(* Logix 5000 AddOnInstructionDefinition export Banner_DFG2_DFG3_Param_v4; software revision 33.00 *)

TYPE Banner_DFG2_DFG3_RD_v4 :   // UDT with all of the Read only parameters for DFG2 or DFG3.
STRUCT
   Master_Cycle_Time : INT;
   Min_Cycle_Time : INT;
   M_Sequence_Capability : INT;
   IO_Link_Version_ID : INT;
   Process_Data_Input_Length : INT;
   Process_Data_Output_Length : INT;
   Combined_Vendor_ID : DINT;   // IO-Link Vendor ID
   Vendor_ID1 : INT;
   Vendor_ID2 : INT;
   Combined_Device_ID : DINT;   // IO-Link Device ID
   Device_ID1 : INT;
   Device_ID2 : INT;
   Device_ID3 : INT;
   Serial_Number : STRING;
   Teach_State : SINT;   // 0 =IDLE, 1 = SP1 Success, 4 = Wait for Command, 5 = Busy, 7 = Error
   SP1_TP1 : SINT;   // 0 = Teach point 1 not taught or not successful, 1 = Teach point 1 was successful
   SP1_TP2 : SINT;   // 0 = Teach point 2 not taught or not successful, 1 = Teach point 2 was successful
   SP2_TP1 : SINT;   // 0 = Teach point 2 not taught or not successful, 1 = Teach point 2 was successful
   SP2_TP2 : SINT;   // 0 = Teach point 2 not taught or not successful, 1 = Teach point 2 was successful
   BDC1_Lower_Hysteresis : DINT;
   BDC1_Lower_Threshold : DINT;
   BDC1_Reference : DINT;
   BDC1_Upper_Threshold : DINT;
   BDC1_Upper_Hysteresis : DINT;
   BDC1_Output_State : SINT;   // 0 = Inactive, 1 = Active.
   BDC1_Alarm_State : SINT;   // 0 = No Alarm, 1 = Threshold Warning, 2 = Threshold Alarm.
   BDC2_Lower_Hysteresis : DINT;
   BDC2_Lower_Threshold : DINT;
   BDC2_Reference : DINT;
   BDC2_Upper_Threshold : DINT;
   BDC2_Upper_Hysteresis : DINT;
   BDC2_Output_State : SINT;   // 0 = Inactive, 1 = Active.
   BDC2_Alarm_State : SINT;   // 0 = No Alarm, 1 = Threshold Warning, 2 = Threshold Alarm.
END_STRUCT
END_TYPE

TYPE Banner_DFG2_DFG3_v4 :   // UDT with all of the parameters needed to work with a Banner DF-G2 or DF-G3 IO-Link Sensor.
STRUCT
   Initial_Global_Read : BOOL;   // Determines if all of the IO-Link data has been read into the PLC yet
   Command : INT;   // Value placed in here will activate a read or write to a specifc IO-Link Index
   DFG_Model : SINT;   // 2 = DF-G2, 3 = DF-G3
   Read_Data : Banner_DFG2_DFG3_RD_v4;
   Write_Data : Banner_DFG2_DFG3_WD_v4;
   Archive_Data : Banner_DFG2_DFG3_WD_v4;
   Reset : BOOL;   // Resets AOI. This will force a complete parameter read of the sensor.
END_STRUCT
END_TYPE

TYPE Banner_DFG2_DFG3_WD_v4 :   // UDT with all of the Write only parameters for DFG2 or DFG3.
STRUCT
   System_Command : INT;   // See IODD file for list of commands that can be activated via the System Command interface
   Parameter_Access_Lock : SINT;   // Write access to all read/write parameters is block when this bit is ON.
   Data_Storage_Lock : SINT;   // Data storage mechanism is inhibited when bit is ON.
   Local_Parameterization_Lock : SINT;   // Parameteriation via local control elementes is inhibited.
   Local_User_Interface_Lock : SINT;   // Operation of the hmi on the device is disabled.
   Teach_Channel : INT;   // 0 = Default, 1 = BDC1, 2 = BDC2
   BDC1_Setpoint_SP1 : DINT;   // Switch point value
   BDC1_Setpoint_SP2 : DINT;   // Unused
   BDC1_Swithpoint_Logic : INT;   // 0 = Light Operate, 1 = Dark Operate
   BDC1_BDC_Mode : INT;   // 1 = Single Point, 128 = Window Set, 129 = Light Set, 130 = Dark Set
   BDC1_Hysteresis : DINT;   // User selectable Hysteresis. 0 = 1.0x, 1 = 1.5x, and 2 = 2.5x.
   BDC2_Setpoint_SP1 : DINT;   // Switch point value
   BDC2_Setpoint_SP2 : DINT;   // Unused
   BDC2_Switchpoint_Logic : INT;   // 0 = Light Operate, 1 = Dark Operate
   BDC2_BDC_Mode : INT;   // 1 = Single Point, 128 = Window Set, 129 = Light Set, 130 = Dark Set
   BDC2_Hysteresis : DINT;   // User selectable Hysteresis. 0 = 1.0x, 1 = 1.5x, and 2 = 2.5x.
   Response_Speed : INT;   // See IODD file for allowable values.
   Gain : INT;   // 0 = Fixed Gain, 1 = Auto Gain
   Gain_Level : INT;   // See IODD file for allowable values.
   AutoThreshold_Response_Time : INT;   // Used in Light, Dark, or Window Set modes only. 12 = 2.5 s, 13 = 5.0 s, 14 = 10 s, and 15 = 20 s.
   Process_Data_Filter_Update_Time : DINT;   // Amount of time to collect averaged sample for process data.
   Signal_Threshold_Readout : INT;   // 0 = Numeric, 1 = Percentage.
   ECO_Mode : INT;   // Dims the display to reduce current consumption. 0 = Disabled, 1 = Enabled.
   Display_Orientation : INT;   // 0 = Normal, 1 = Flipped.
   Secondary_Output_Function : INT;   // 0 = Independent Output, 1 = Complimentary Output, 2 = Health Output, 3 = Remote Set Input, 4 = Master, 5 = Slave, 6 = LED Off, 7 = LED On, 8 = Gate.
   Slave_Numder : INT;   // Total slaves presetn if in master mode. Slave Address if configured as slave. 1 to 6.
   BDC1_Delay_Mode : INT;   // 0 = Disabled, 1 = Off - On Delay, 2 = Off Oneshot, 3 = On Oneshot
   BDC1_Delay_Timer1 : DINT;   // 0 to 9999. Off delay or On/Off Oneshot time. If configured in Oneshot mode, this parameter wil have a minimum value of 1 ms.
   BDC1_Delay_Timer2 : DINT;   // 0 to 9999. On delay time or additional delay time. In off/on delay mode, this parameter will be the on delay.
   BDC1_Teach_Selection : INT;   // 0 = Two-Point Teach, 1 = Dynamic Teach, 2 = Window Teach, 3 = Light Set, 4 = Dark Set, 5 = Cal Set
   BDC1_Offset_Percent : DINT;   // Used during the Window, Light, or Dark Set methods. The threshold(s) are positioned in a programmable % offset from the taught condition.
   BDC1_Auto_Thresholding : INT;   // 0 = Disabled, 1 = Enabled. The auto thresholds algorithm continuously tracks slow changes in the taught condition(s) and optimizes the threshold(s) to provide for reliable sensing.
   BDC2_Delay_Mode : INT;   // 0 = Disabled, 1 = Off - On Delay, 2 = Off Oneshot, 3 = On Oneshot
   BDC2_Delay_Timer1 : DINT;   // 0 to 9999. Off delay or On/Off Oneshot time. If configured in Oneshot mode, this parameter wil have a minimum value of 1 ms.
   BDC2_Delay_Timer2 : DINT;   // 0 to 9999. On delay time or additional delay time. In off/on delay mode, this parameter will be the on delay.
   BDC2_Teach_Selection : INT;   // 0 = Two-Point Teach, 1 = Dynamic Teach, 2 = Window Teach, 3 = Light Set, 4 = Dark Set, 5 = Cal Set
   BDC2_Offset_Percent : DINT;   // Used during the Window, Light, or Dark Set methods. The threshold(s) are positioned in a programmable % offset from the taught condition.
   BDC2_Auto_Thresholding : INT;   // 0 = Disabled, 1 = Enabled. The auto thresholds algorithm continuously tracks slow changes in the taught condition(s) and optimizes the threshold(s) to provide for reliable sensing.
END_STRUCT
END_TYPE

TYPE Banner_IOL_Port_v4 :   // UDT that has all of the data items necessary to communicate with a specific Port on a IO-Link Master
STRUCT
   Port_Controlled : INT;   // Each bit represents a port on an IO-Link Master. Set to 1 to tell AOI to control that port.
   Port_Activate : INT;   // Each bit represents a port on an IO-Link Master. When ON that port will process any commands in queue.
   Port_Read : INT;   // Each bit represents a port on an IO-Link Master. Used to determine when device AOI has requested a Read command.
   Port_Write : INT;   // Each bit represents a port on an IO-Link Master. Used to determine when device AOI has requested a Write command.
   Port_RW_Complete : INT;   // Each bit represents a port on an IO-Link Master. Tells device AOI that Read or Write request has been completed.
   Port_Device_Read : INT;
   Data_Transfer : SINT[190];   // Array to transfer data from IO-Master to device AOIs.
END_STRUCT
END_TYPE

ADD_ON_INSTRUCTION Banner_DFG2_DFG3_Param_v4   (* revision 4.1, vendor Banner Engineering *)
// AOI to read and write parameter data to an IO-Link Df-G2 or DF-G3.
VAR_IN_OUT
   DFG2_DFG3 : Banner_DFG2_DFG3_v4; {required}
   Port_Data : Banner_IOL_Port_v4; {required}
END_VAR
VAR_INPUT
   Port : DINT; {required}
END_VAR
VAR
   Local_Control : DINT; {access None}
   Global_Read_Command_Value : INT; {access None}
   Global_Write_Command_Value : INT; {access None}
   Error_Generated : BOOL; {access None}
   Command_Being_Processed : BOOL; {access None}
   Update_Archive : BOOL; {access None}
   Index_Write_Inprocess : DINT; {access None}
   Index_Write_Control : DINT; {access None}
   Inprocess_Index : DINT; {access None}
END_VAR

ROUTINE Logic   (* ladder *)
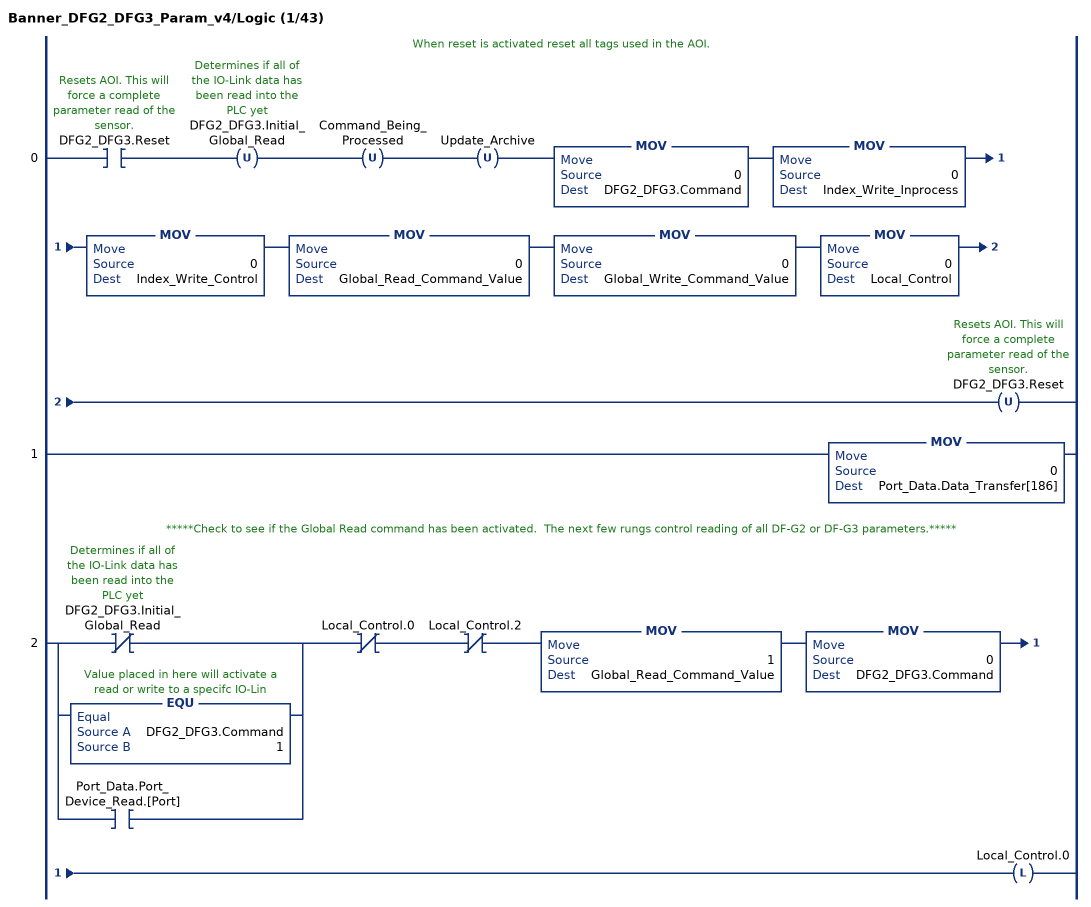
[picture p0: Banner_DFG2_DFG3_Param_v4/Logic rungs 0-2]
   // When reset is activated reset all tags used in the AOI.
   0: XIC(DFG2_DFG3.Reset)OTU(DFG2_DFG3.Initial_Global_Read)OTU(Command_Being_Processed)OTU(Update_Archive)MOV(0,DFG2_DFG3.Command)MOV(0,Index_Write_Inprocess)MOV(0,Index_Write_Control)MOV(0,Global_Read_Command_Value)MOV(0,Global_Write_Command_Value)MOV(0,Local_Control)OTU(DFG2_DFG3.Reset);
   1: MOV(0,Port_Data.Data_Transfer[186]);
   // *****Check to see if the Global Read command has been activated.  The next few rungs control reading of all DF-G2 or DF-G3 parameters.*****
   2: [XIO(DFG2_DFG3.Initial_Global_Read) ,EQU(DFG2_DFG3.Command,1) ,XIC(Port_Data.Port_Device_Read.[Port]) ]XIO(Local_Control.0)XIO(Local_Control.2)MOV(1,Global_Read_Command_Value)MOV(0,DFG2_DFG3.Command)OTL(Local_Control.0);
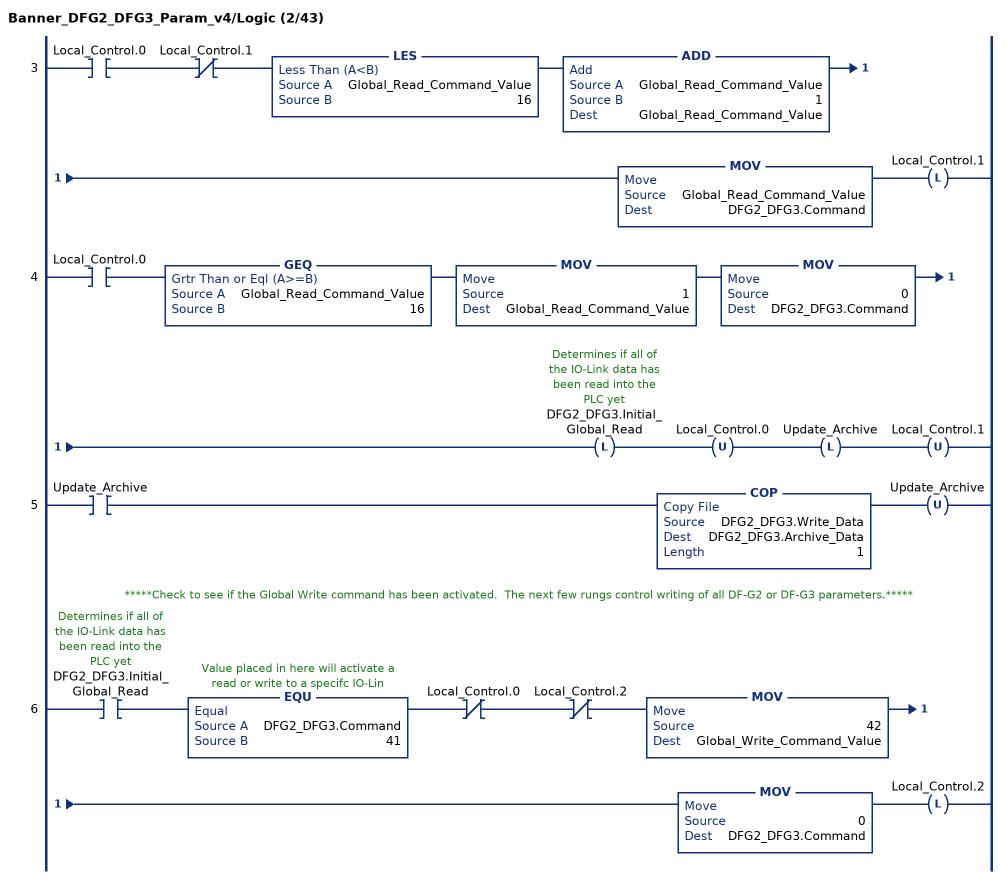
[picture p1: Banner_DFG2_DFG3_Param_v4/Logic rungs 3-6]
   3: XIC(Local_Control.0)XIO(Local_Control.1)LES(Global_Read_Command_Value,16)ADD(Global_Read_Command_Value,1,Global_Read_Command_Value)MOV(Global_Read_Command_Value,DFG2_DFG3.Command)OTL(Local_Control.1);
   4: XIC(Local_Control.0)GEQ(Global_Read_Command_Value,16)MOV(1,Global_Read_Command_Value)MOV(0,DFG2_DFG3.Command)OTL(DFG2_DFG3.Initial_Global_Read)OTU(Local_Control.0)OTL(Update_Archive)OTU(Local_Control.1);
   5: XIC(Update_Archive)COP(DFG2_DFG3.Write_Data,DFG2_DFG3.Archive_Data,1)OTU(Update_Archive);
   // *****Check to see if the Global Write command has been activated.  The next few rungs control writing of all DF-G2 or DF-G3 parameters.*****
   6: XIC(DFG2_DFG3.Initial_Global_Read)EQU(DFG2_DFG3.Command,41)XIO(Local_Control.0)XIO(Local_Control.2)MOV(42,Global_Write_Command_Value)MOV(0,DFG2_DFG3.Command)OTL(Local_Control.2);
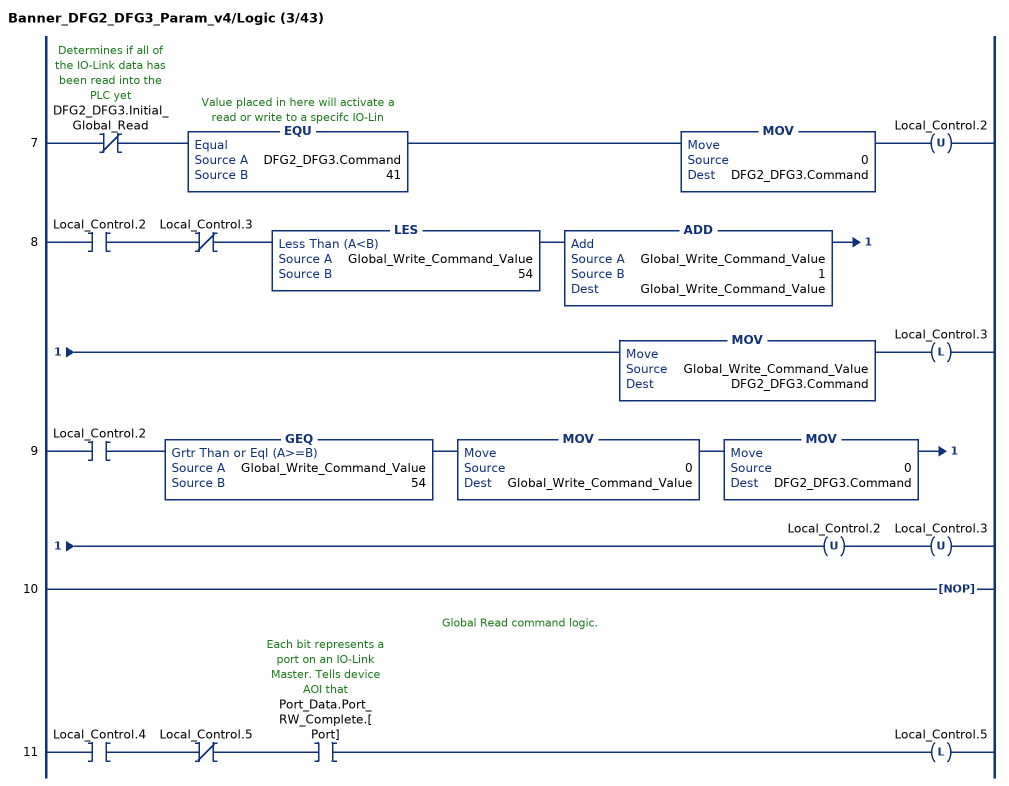
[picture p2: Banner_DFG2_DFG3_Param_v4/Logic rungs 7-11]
   7: XIO(DFG2_DFG3.Initial_Global_Read)EQU(DFG2_DFG3.Command,41)MOV(0,DFG2_DFG3.Command)OTU(Local_Control.2);
   8: XIC(Local_Control.2)XIO(Local_Control.3)LES(Global_Write_Command_Value,54)ADD(Global_Write_Command_Value,1,Global_Write_Command_Value)MOV(Global_Write_Command_Value,DFG2_DFG3.Command)OTL(Local_Control.3);
   9: XIC(Local_Control.2)GEQ(Global_Write_Command_Value,54)MOV(0,Global_Write_Command_Value)MOV(0,DFG2_DFG3.Command)OTU(Local_Control.2)OTU(Local_Control.3);
   10: NOP();
   // Global Read command logic.
   11: XIC(Local_Control.4)XIO(Local_Control.5)XIC(Port_Data.Port_RW_Complete.[Port])OTL(Local_Control.5);
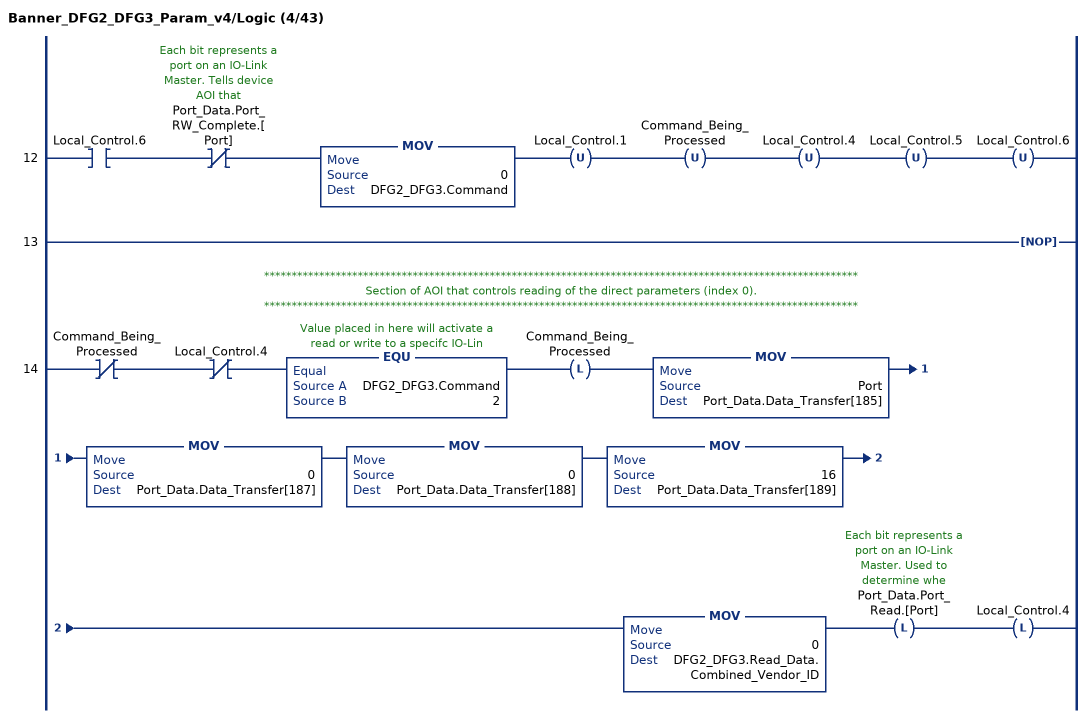
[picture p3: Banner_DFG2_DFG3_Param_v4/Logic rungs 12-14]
   12: XIC(Local_Control.6)XIO(Port_Data.Port_RW_Complete.[Port])MOV(0,DFG2_DFG3.Command)OTU(Local_Control.1)OTU(Command_Being_Processed)OTU(Local_Control.4)OTU(Local_Control.5)OTU(Local_Control.6);
   13: NOP();
   // ************************************************************************************************************
   // Section of AOI that controls reading of the direct parameters (index 0).
   // ************************************************************************************************************
   14: XIO(Command_Being_Processed)XIO(Local_Control.4)EQU(DFG2_DFG3.Command,2)OTL(Command_Being_Processed)MOV(Port,Port_Data.Data_Transfer[185])MOV(0,Port_Data.Data_Transfer[187])MOV(0,Port_Data.Data_Transfer[188])MOV(16,Port_Data.Data_Transfer[189])MOV(0,DFG2_DFG3.Read_Data.Combined_Vendor_ID)OTL(Port_Data.Port_Read.[Port])OTL(Local_Control.4);
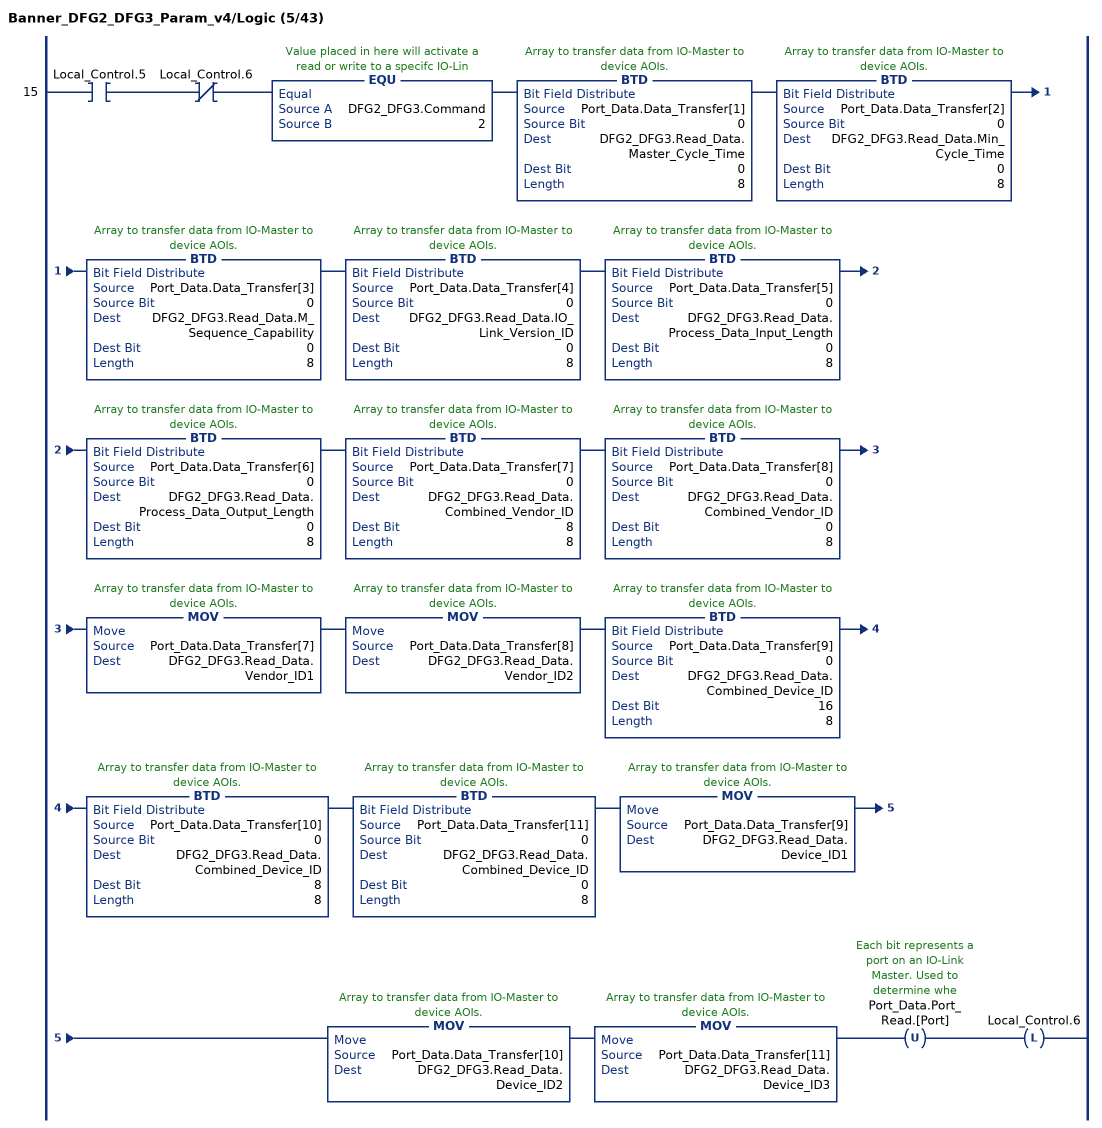
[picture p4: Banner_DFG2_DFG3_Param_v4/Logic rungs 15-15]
   15: XIC(Local_Control.5)XIO(Local_Control.6)EQU(DFG2_DFG3.Command,2)BTD(Port_Data.Data_Transfer[1],0,DFG2_DFG3.Read_Data.Master_Cycle_Time,0,8)BTD(Port_Data.Data_Transfer[2],0,DFG2_DFG3.Read_Data.Min_Cycle_Time,0,8)BTD(Port_Data.Data_Transfer[3],0,DFG2_DFG3.Read_Data.M_Sequence_Capability,0,8)BTD(Port_Data.Data_Transfer[4],0,DFG2_DFG3.Read_Data.IO_Link_Version_ID,0,8)BTD(Port_Data.Data_Transfer[5],0,DFG2_DFG3.Read_Data.Process_Data_Input_Length,0,8)BTD(Port_Data.Data_Transfer[6],0,DFG2_DFG3.Read_Data.Process_Data_Output_Length,0,8)BTD(Port_Data.Data_Transfer[7],0,DFG2_DFG3.Read_Data.Combined_Vendor_ID,8,8)BTD(Port_Data.Data_Transfer[8],0,DFG2_DFG3.Read_Data.Combined_Vendor_ID,0,8)MOV(Port_Data.Data_Transfer[7],DFG2_DFG3.Read_Data.Vendor_ID1)MOV(Port_Data.Data_Transfer[8],DFG2_DFG3.Read_Data.Vendor_ID2)BTD(Port_Data.Data_Transfer[9],0,DFG2_DFG3.Read_Data.Combined_Device_ID,16,8)BTD(Port_Data.Data_Transfer[10],0,DFG2_DFG3.Read_Data.Combined_Device_ID,8,8)BTD(Port_Data.Data_Transfer[11],0,DFG2_DFG3.Read_Data.Combined_Device_ID,0,8)MOV(Port_Data.Data_Transfer[9],DFG2_DFG3.Read_Data.Device_ID1)MOV(Port_Data.Data_Transfer[10],DFG2_DFG3.Read_Data.Device_ID2)MOV(Port_Data.Data_Transfer[11],DFG2_DFG3.Read_Data.Device_ID3)OTU(Port_Data.Port_Read.[Port])OTL(Local_Control.6);
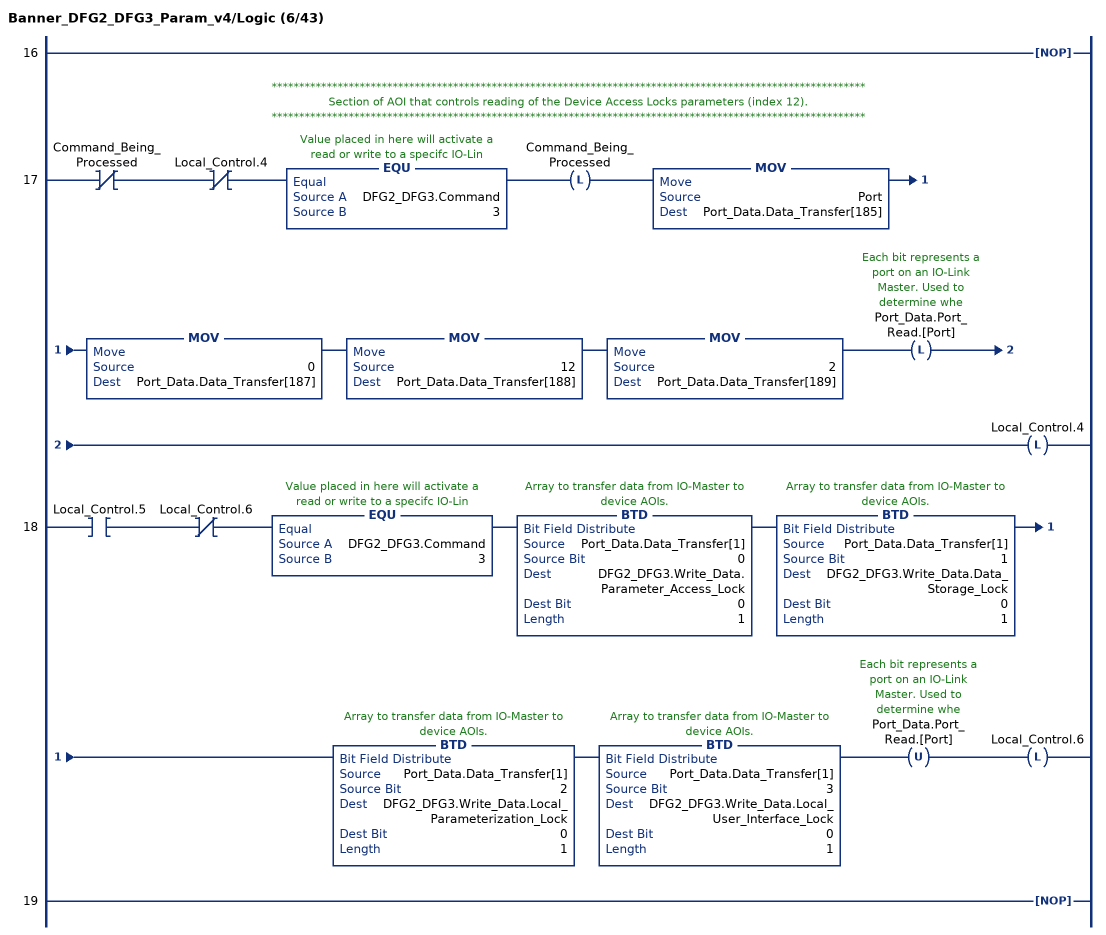
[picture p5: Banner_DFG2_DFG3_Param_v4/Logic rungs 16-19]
   16: NOP();
   // ************************************************************************************************************
   // Section of AOI that controls reading of the Device Access Locks parameters (index 12).
   // ************************************************************************************************************
   17: XIO(Command_Being_Processed)XIO(Local_Control.4)EQU(DFG2_DFG3.Command,3)OTL(Command_Being_Processed)MOV(Port,Port_Data.Data_Transfer[185])MOV(0,Port_Data.Data_Transfer[187])MOV(12,Port_Data.Data_Transfer[188])MOV(2,Port_Data.Data_Transfer[189])OTL(Port_Data.Port_Read.[Port])OTL(Local_Control.4);
   18: XIC(Local_Control.5)XIO(Local_Control.6)EQU(DFG2_DFG3.Command,3)BTD(Port_Data.Data_Transfer[1],0,DFG2_DFG3.Write_Data.Parameter_Access_Lock,0,1)BTD(Port_Data.Data_Transfer[1],1,DFG2_DFG3.Write_Data.Data_Storage_Lock,0,1)BTD(Port_Data.Data_Transfer[1],2,DFG2_DFG3.Write_Data.Local_Parameterization_Lock,0,1)BTD(Port_Data.Data_Transfer[1],3,DFG2_DFG3.Write_Data.Local_User_Interface_Lock,0,1)OTU(Port_Data.Port_Read.[Port])OTL(Local_Control.6);
   19: NOP();
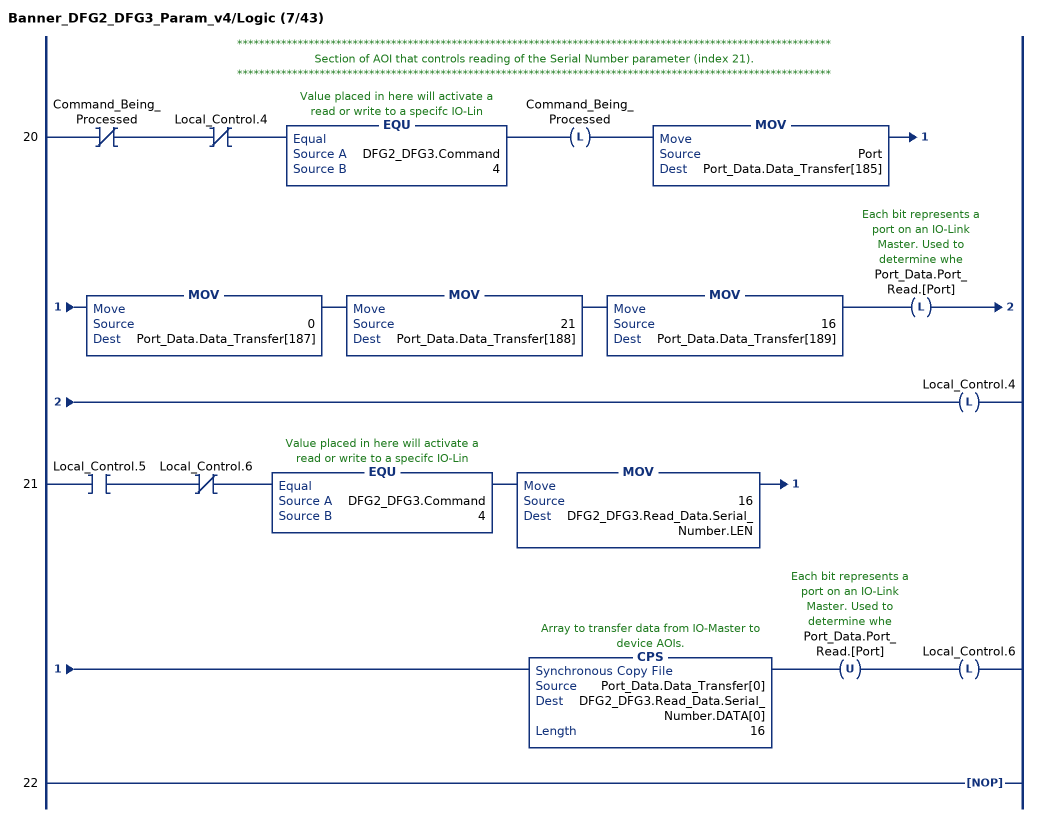
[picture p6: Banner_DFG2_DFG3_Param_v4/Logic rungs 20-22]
   // ************************************************************************************************************
   // Section of AOI that controls reading of the Serial Number parameter (index 21).
   // ************************************************************************************************************
   20: XIO(Command_Being_Processed)XIO(Local_Control.4)EQU(DFG2_DFG3.Command,4)OTL(Command_Being_Processed)MOV(Port,Port_Data.Data_Transfer[185])MOV(0,Port_Data.Data_Transfer[187])MOV(21,Port_Data.Data_Transfer[188])MOV(16,Port_Data.Data_Transfer[189])OTL(Port_Data.Port_Read.[Port])OTL(Local_Control.4);
   21: XIC(Local_Control.5)XIO(Local_Control.6)EQU(DFG2_DFG3.Command,4)MOV(16,DFG2_DFG3.Read_Data.Serial_Number.LEN)CPS(Port_Data.Data_Transfer[0],DFG2_DFG3.Read_Data.Serial_Number.DATA[0],16)OTU(Port_Data.Port_Read.[Port])OTL(Local_Control.6);
   22: NOP();
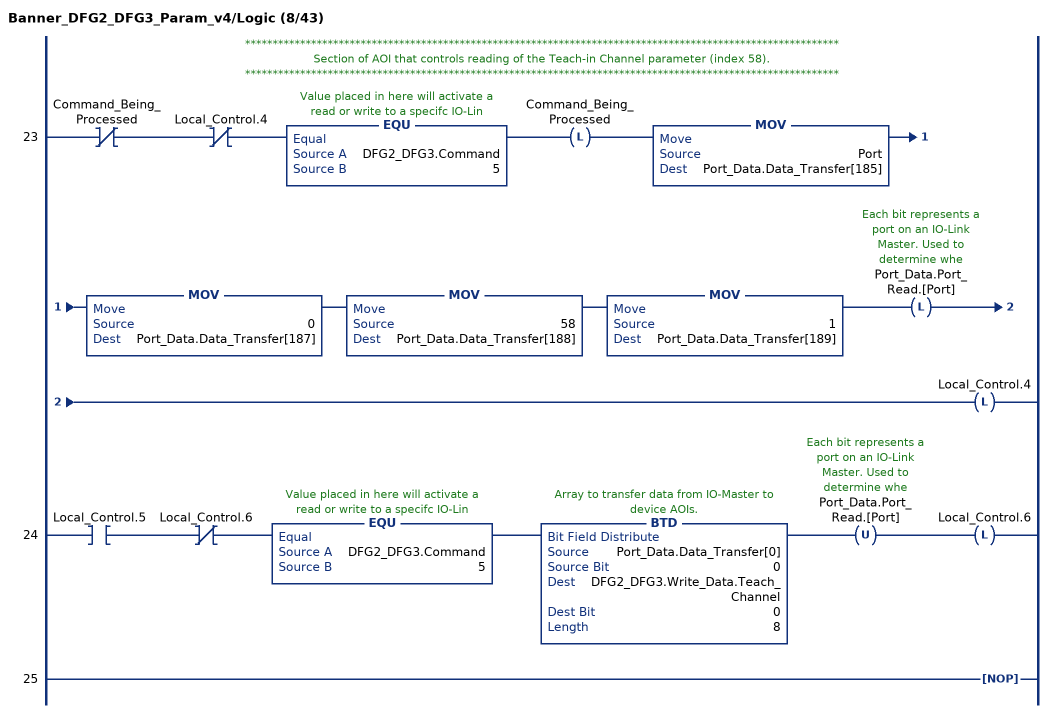
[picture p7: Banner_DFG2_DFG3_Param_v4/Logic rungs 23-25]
   // ************************************************************************************************************
   // Section of AOI that controls reading of the Teach-in Channel parameter (index 58).
   // ************************************************************************************************************
   23: XIO(Command_Being_Processed)XIO(Local_Control.4)EQU(DFG2_DFG3.Command,5)OTL(Command_Being_Processed)MOV(Port,Port_Data.Data_Transfer[185])MOV(0,Port_Data.Data_Transfer[187])MOV(58,Port_Data.Data_Transfer[188])MOV(1,Port_Data.Data_Transfer[189])OTL(Port_Data.Port_Read.[Port])OTL(Local_Control.4);
   24: XIC(Local_Control.5)XIO(Local_Control.6)EQU(DFG2_DFG3.Command,5)BTD(Port_Data.Data_Transfer[0],0,DFG2_DFG3.Write_Data.Teach_Channel,0,8)OTU(Port_Data.Port_Read.[Port])OTL(Local_Control.6);
   25: NOP();
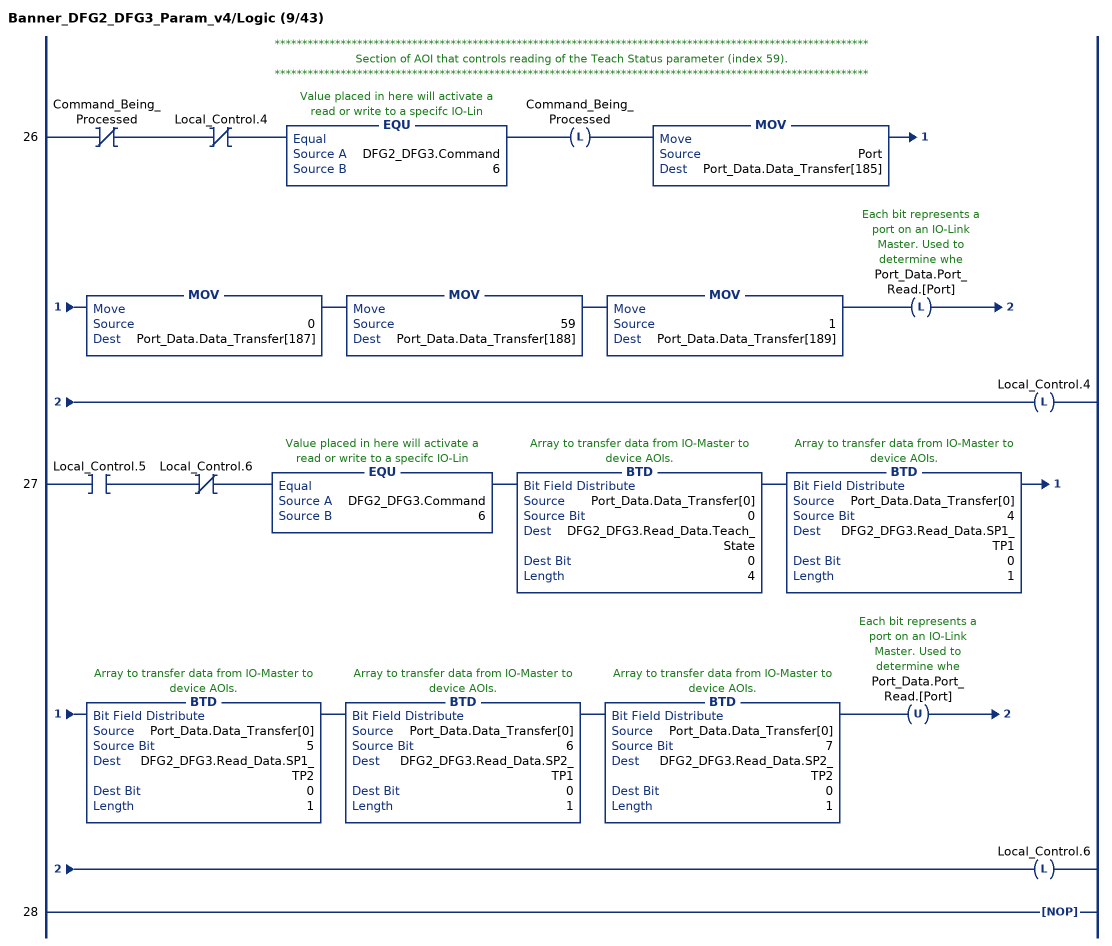
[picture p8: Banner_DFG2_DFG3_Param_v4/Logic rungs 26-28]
   // ************************************************************************************************************
   // Section of AOI that controls reading of the Teach Status parameter (index 59).
   // ************************************************************************************************************
   26: XIO(Command_Being_Processed)XIO(Local_Control.4)EQU(DFG2_DFG3.Command,6)OTL(Command_Being_Processed)MOV(Port,Port_Data.Data_Transfer[185])MOV(0,Port_Data.Data_Transfer[187])MOV(59,Port_Data.Data_Transfer[188])MOV(1,Port_Data.Data_Transfer[189])OTL(Port_Data.Port_Read.[Port])OTL(Local_Control.4);
   27: XIC(Local_Control.5)XIO(Local_Control.6)EQU(DFG2_DFG3.Command,6)BTD(Port_Data.Data_Transfer[0],0,DFG2_DFG3.Read_Data.Teach_State,0,4)BTD(Port_Data.Data_Transfer[0],4,DFG2_DFG3.Read_Data.SP1_TP1,0,1)BTD(Port_Data.Data_Transfer[0],5,DFG2_DFG3.Read_Data.SP1_TP2,0,1)BTD(Port_Data.Data_Transfer[0],6,DFG2_DFG3.Read_Data.SP2_TP1,0,1)BTD(Port_Data.Data_Transfer[0],7,DFG2_DFG3.Read_Data.SP2_TP2,0,1)OTU(Port_Data.Port_Read.[Port])OTL(Local_Control.6);
   28: NOP();
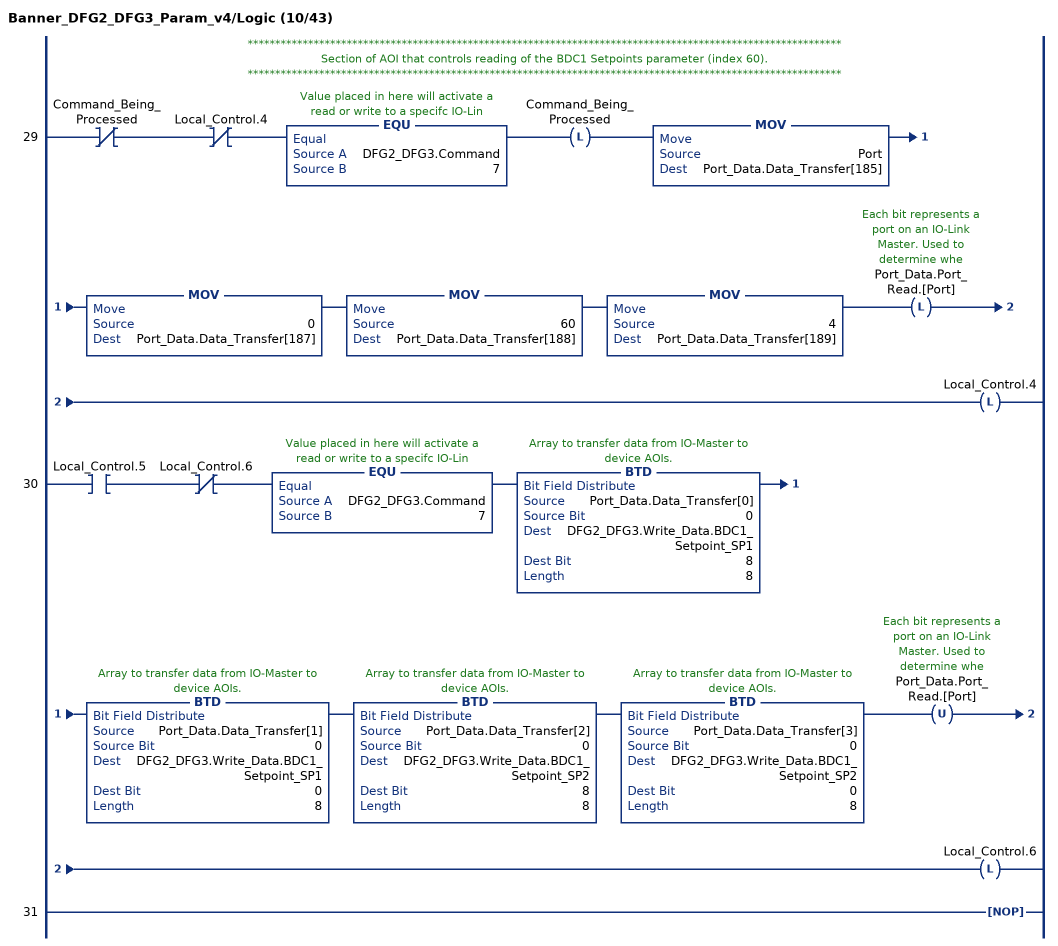
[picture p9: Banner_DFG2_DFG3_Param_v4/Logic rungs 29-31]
   // ************************************************************************************************************
   // Section of AOI that controls reading of the BDC1 Setpoints parameter (index 60).
   // ************************************************************************************************************
   29: XIO(Command_Being_Processed)XIO(Local_Control.4)EQU(DFG2_DFG3.Command,7)OTL(Command_Being_Processed)MOV(Port,Port_Data.Data_Transfer[185])MOV(0,Port_Data.Data_Transfer[187])MOV(60,Port_Data.Data_Transfer[188])MOV(4,Port_Data.Data_Transfer[189])OTL(Port_Data.Port_Read.[Port])OTL(Local_Control.4);
   30: XIC(Local_Control.5)XIO(Local_Control.6)EQU(DFG2_DFG3.Command,7)BTD(Port_Data.Data_Transfer[0],0,DFG2_DFG3.Write_Data.BDC1_Setpoint_SP1,8,8)BTD(Port_Data.Data_Transfer[1],0,DFG2_DFG3.Write_Data.BDC1_Setpoint_SP1,0,8)BTD(Port_Data.Data_Transfer[2],0,DFG2_DFG3.Write_Data.BDC1_Setpoint_SP2,8,8)BTD(Port_Data.Data_Transfer[3],0,DFG2_DFG3.Write_Data.BDC1_Setpoint_SP2,0,8)OTU(Port_Data.Port_Read.[Port])OTL(Local_Control.6);
   31: NOP();
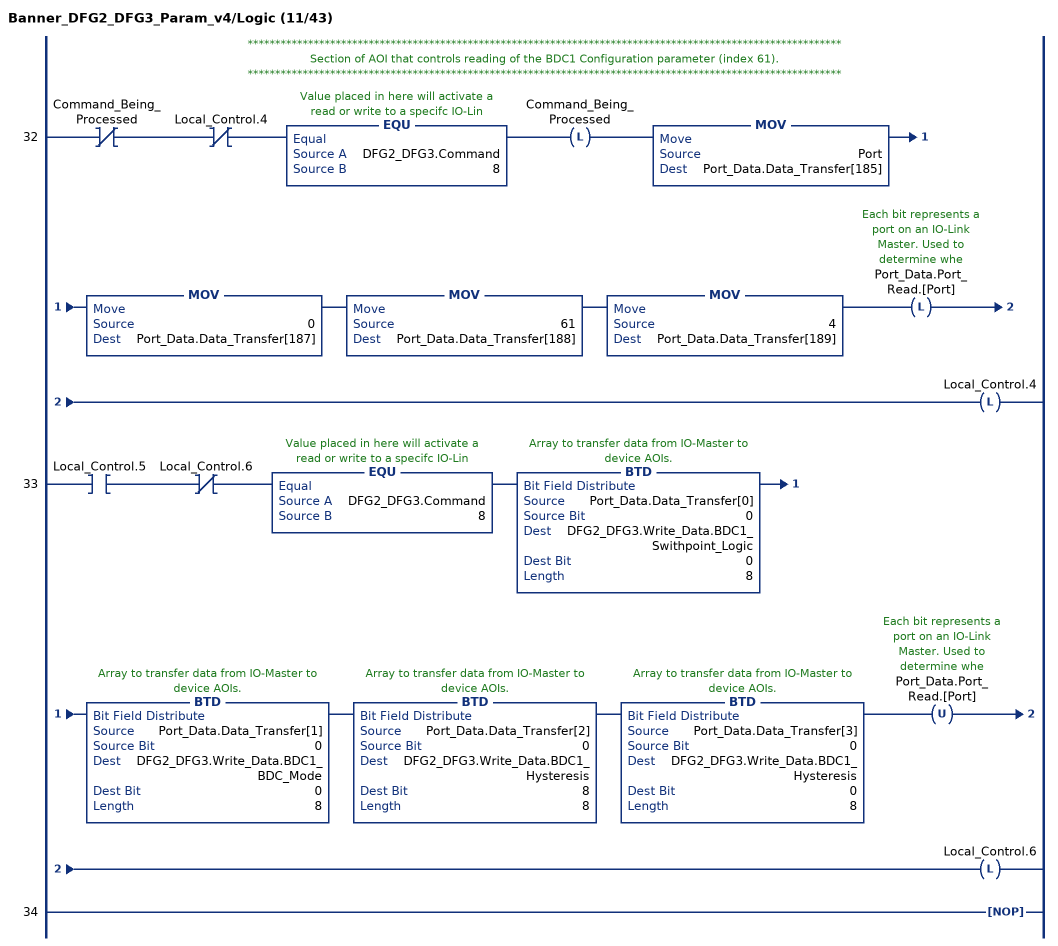
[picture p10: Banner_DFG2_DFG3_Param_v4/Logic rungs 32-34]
   // ************************************************************************************************************
   // Section of AOI that controls reading of the BDC1 Configuration parameter (index 61).
   // ************************************************************************************************************
   32: XIO(Command_Being_Processed)XIO(Local_Control.4)EQU(DFG2_DFG3.Command,8)OTL(Command_Being_Processed)MOV(Port,Port_Data.Data_Transfer[185])MOV(0,Port_Data.Data_Transfer[187])MOV(61,Port_Data.Data_Transfer[188])MOV(4,Port_Data.Data_Transfer[189])OTL(Port_Data.Port_Read.[Port])OTL(Local_Control.4);
   33: XIC(Local_Control.5)XIO(Local_Control.6)EQU(DFG2_DFG3.Command,8)BTD(Port_Data.Data_Transfer[0],0,DFG2_DFG3.Write_Data.BDC1_Swithpoint_Logic,0,8)BTD(Port_Data.Data_Transfer[1],0,DFG2_DFG3.Write_Data.BDC1_BDC_Mode,0,8)BTD(Port_Data.Data_Transfer[2],0,DFG2_DFG3.Write_Data.BDC1_Hysteresis,8,8)BTD(Port_Data.Data_Transfer[3],0,DFG2_DFG3.Write_Data.BDC1_Hysteresis,0,8)OTU(Port_Data.Port_Read.[Port])OTL(Local_Control.6);
   34: NOP();
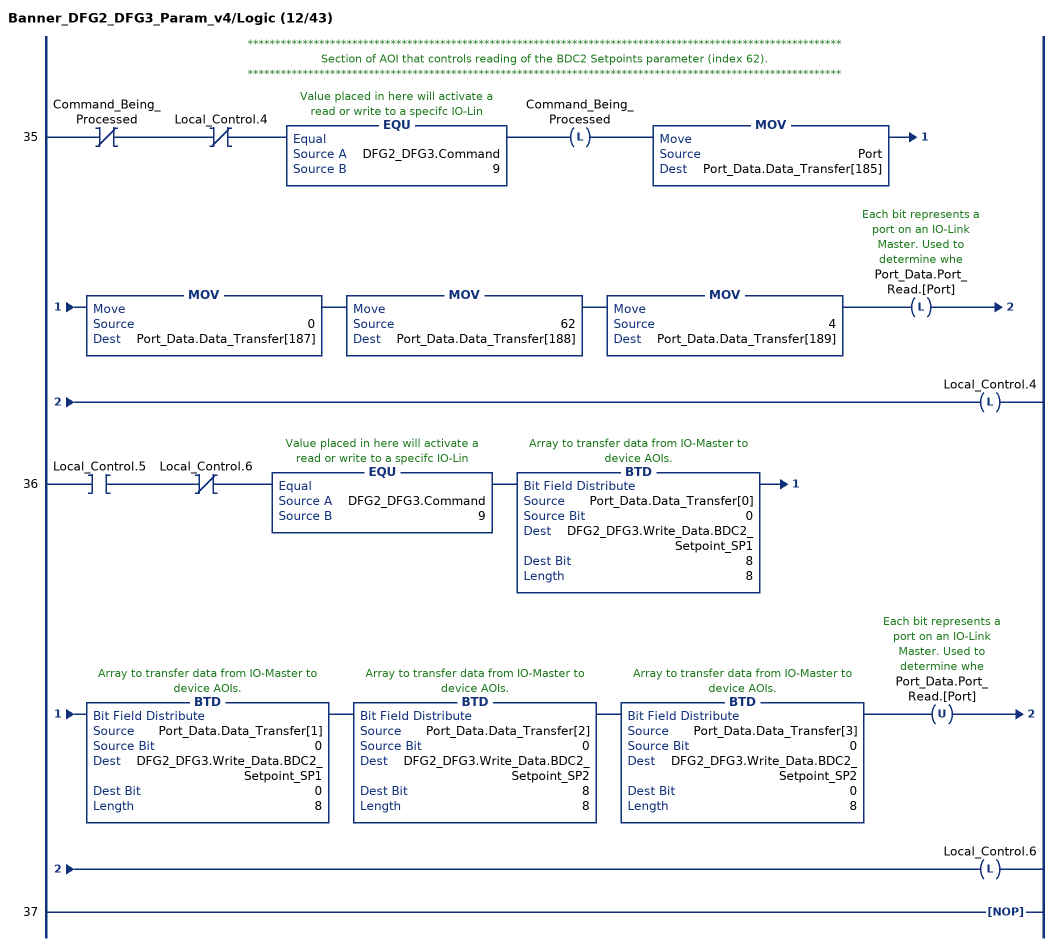
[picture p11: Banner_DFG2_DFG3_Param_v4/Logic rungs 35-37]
   // ************************************************************************************************************
   // Section of AOI that controls reading of the BDC2 Setpoints parameter (index 62).
   // ************************************************************************************************************
   35: XIO(Command_Being_Processed)XIO(Local_Control.4)EQU(DFG2_DFG3.Command,9)OTL(Command_Being_Processed)MOV(Port,Port_Data.Data_Transfer[185])MOV(0,Port_Data.Data_Transfer[187])MOV(62,Port_Data.Data_Transfer[188])MOV(4,Port_Data.Data_Transfer[189])OTL(Port_Data.Port_Read.[Port])OTL(Local_Control.4);
   36: XIC(Local_Control.5)XIO(Local_Control.6)EQU(DFG2_DFG3.Command,9)BTD(Port_Data.Data_Transfer[0],0,DFG2_DFG3.Write_Data.BDC2_Setpoint_SP1,8,8)BTD(Port_Data.Data_Transfer[1],0,DFG2_DFG3.Write_Data.BDC2_Setpoint_SP1,0,8)BTD(Port_Data.Data_Transfer[2],0,DFG2_DFG3.Write_Data.BDC2_Setpoint_SP2,8,8)BTD(Port_Data.Data_Transfer[3],0,DFG2_DFG3.Write_Data.BDC2_Setpoint_SP2,0,8)OTU(Port_Data.Port_Read.[Port])OTL(Local_Control.6);
   37: NOP();
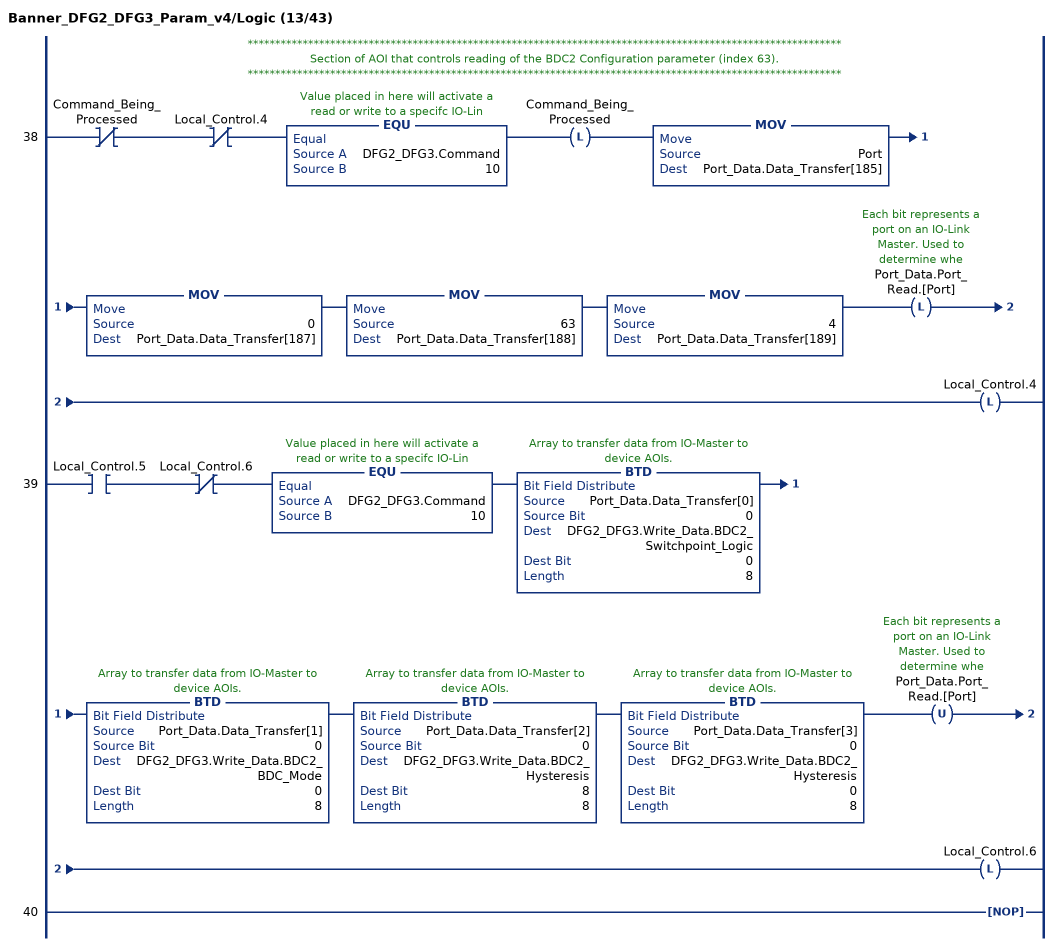
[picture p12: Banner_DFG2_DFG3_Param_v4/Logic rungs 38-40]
   // ************************************************************************************************************
   // Section of AOI that controls reading of the BDC2 Configuration parameter (index 63).
   // ************************************************************************************************************
   38: XIO(Command_Being_Processed)XIO(Local_Control.4)EQU(DFG2_DFG3.Command,10)OTL(Command_Being_Processed)MOV(Port,Port_Data.Data_Transfer[185])MOV(0,Port_Data.Data_Transfer[187])MOV(63,Port_Data.Data_Transfer[188])MOV(4,Port_Data.Data_Transfer[189])OTL(Port_Data.Port_Read.[Port])OTL(Local_Control.4);
   39: XIC(Local_Control.5)XIO(Local_Control.6)EQU(DFG2_DFG3.Command,10)BTD(Port_Data.Data_Transfer[0],0,DFG2_DFG3.Write_Data.BDC2_Switchpoint_Logic,0,8)BTD(Port_Data.Data_Transfer[1],0,DFG2_DFG3.Write_Data.BDC2_BDC_Mode,0,8)BTD(Port_Data.Data_Transfer[2],0,DFG2_DFG3.Write_Data.BDC2_Hysteresis,8,8)BTD(Port_Data.Data_Transfer[3],0,DFG2_DFG3.Write_Data.BDC2_Hysteresis,0,8)OTU(Port_Data.Port_Read.[Port])OTL(Local_Control.6);
   40: NOP();
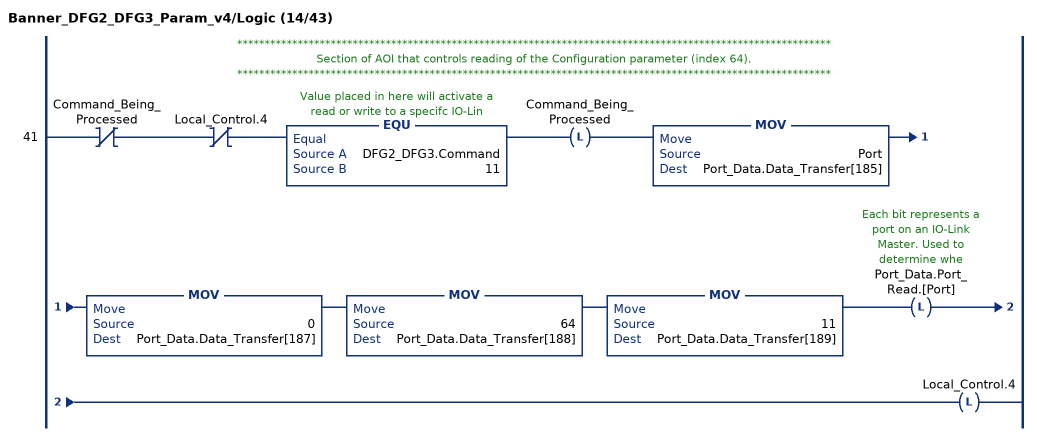
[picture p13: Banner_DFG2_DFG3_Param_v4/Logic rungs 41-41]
   // ************************************************************************************************************
   // Section of AOI that controls reading of the Configuration parameter (index 64).
   // ************************************************************************************************************
   41: XIO(Command_Being_Processed)XIO(Local_Control.4)EQU(DFG2_DFG3.Command,11)OTL(Command_Being_Processed)MOV(Port,Port_Data.Data_Transfer[185])MOV(0,Port_Data.Data_Transfer[187])MOV(64,Port_Data.Data_Transfer[188])MOV(11,Port_Data.Data_Transfer[189])OTL(Port_Data.Port_Read.[Port])OTL(Local_Control.4);
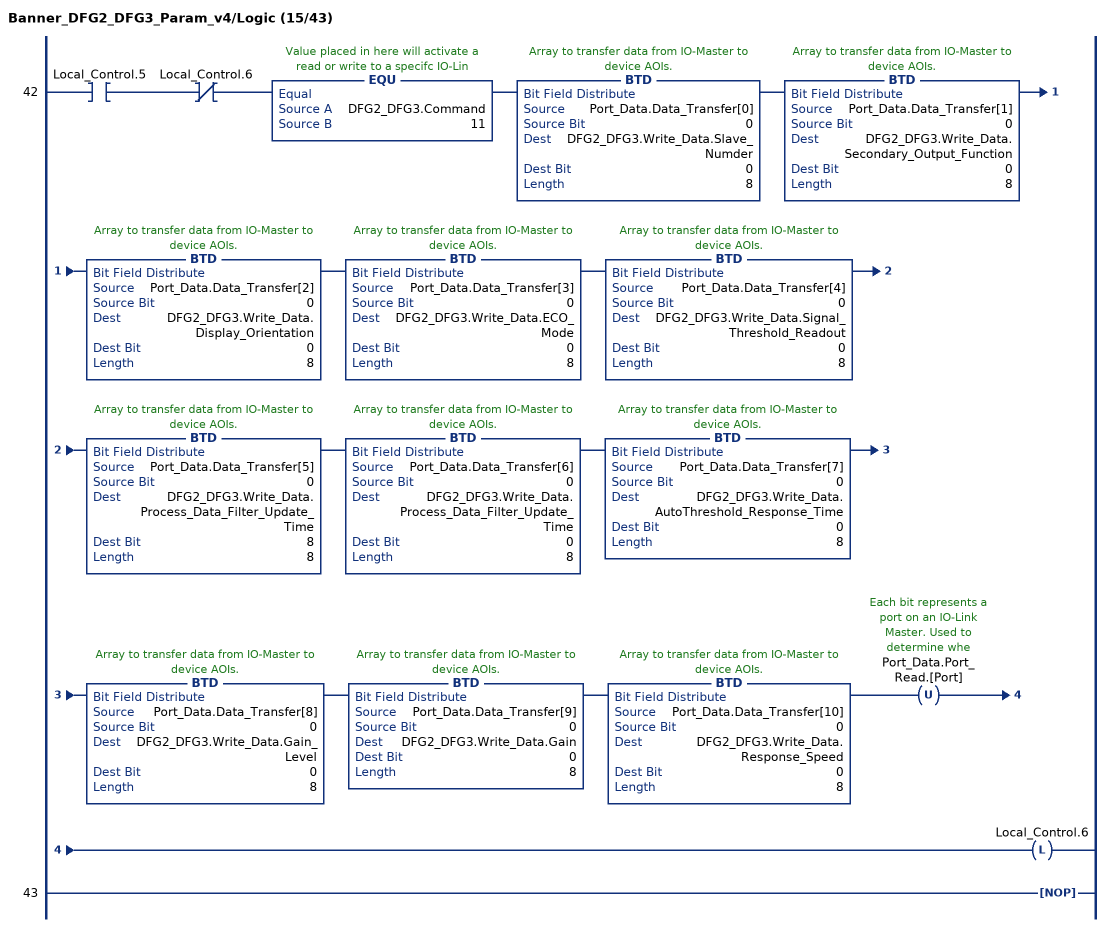
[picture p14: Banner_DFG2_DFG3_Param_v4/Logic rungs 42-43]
   42: XIC(Local_Control.5)XIO(Local_Control.6)EQU(DFG2_DFG3.Command,11)BTD(Port_Data.Data_Transfer[0],0,DFG2_DFG3.Write_Data.Slave_Numder,0,8)BTD(Port_Data.Data_Transfer[1],0,DFG2_DFG3.Write_Data.Secondary_Output_Function,0,8)BTD(Port_Data.Data_Transfer[2],0,DFG2_DFG3.Write_Data.Display_Orientation,0,8)BTD(Port_Data.Data_Transfer[3],0,DFG2_DFG3.Write_Data.ECO_Mode,0,8)BTD(Port_Data.Data_Transfer[4],0,DFG2_DFG3.Write_Data.Signal_Threshold_Readout,0,8)BTD(Port_Data.Data_Transfer[5],0,DFG2_DFG3.Write_Data.Process_Data_Filter_Update_Time,8,8)BTD(Port_Data.Data_Transfer[6],0,DFG2_DFG3.Write_Data.Process_Data_Filter_Update_Time,0,8)BTD(Port_Data.Data_Transfer[7],0,DFG2_DFG3.Write_Data.AutoThreshold_Response_Time,0,8)BTD(Port_Data.Data_Transfer[8],0,DFG2_DFG3.Write_Data.Gain_Level,0,8)BTD(Port_Data.Data_Transfer[9],0,DFG2_DFG3.Write_Data.Gain,0,8)BTD(Port_Data.Data_Transfer[10],0,DFG2_DFG3.Write_Data.Response_Speed,0,8)OTU(Port_Data.Port_Read.[Port])OTL(Local_Control.6);
   43: NOP();
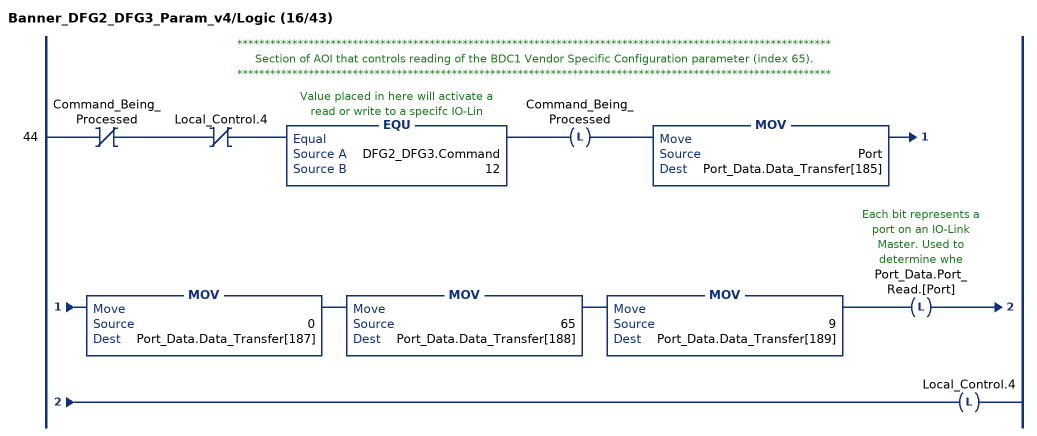
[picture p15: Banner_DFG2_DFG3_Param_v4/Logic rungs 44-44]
   // ************************************************************************************************************
   // Section of AOI that controls reading of the BDC1 Vendor Specific Configuration parameter (index 65).
   // ************************************************************************************************************
   44: XIO(Command_Being_Processed)XIO(Local_Control.4)EQU(DFG2_DFG3.Command,12)OTL(Command_Being_Processed)MOV(Port,Port_Data.Data_Transfer[185])MOV(0,Port_Data.Data_Transfer[187])MOV(65,Port_Data.Data_Transfer[188])MOV(9,Port_Data.Data_Transfer[189])OTL(Port_Data.Port_Read.[Port])OTL(Local_Control.4);
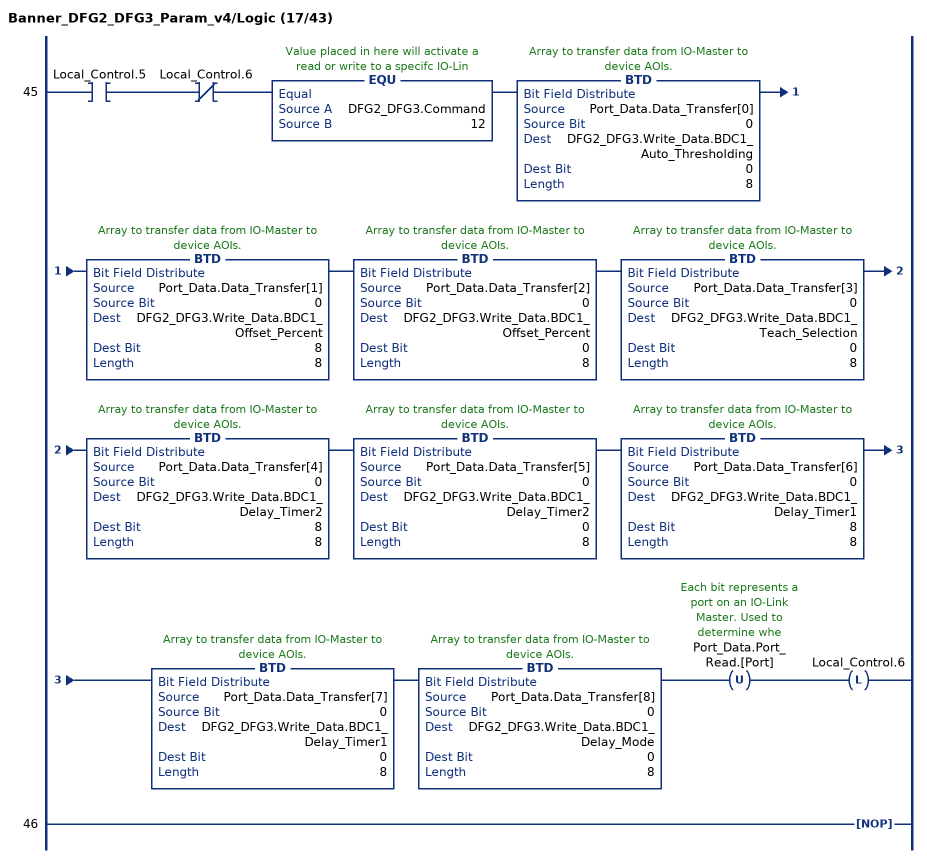
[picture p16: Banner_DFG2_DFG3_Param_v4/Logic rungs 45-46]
   45: XIC(Local_Control.5)XIO(Local_Control.6)EQU(DFG2_DFG3.Command,12)BTD(Port_Data.Data_Transfer[0],0,DFG2_DFG3.Write_Data.BDC1_Auto_Thresholding,0,8)BTD(Port_Data.Data_Transfer[1],0,DFG2_DFG3.Write_Data.BDC1_Offset_Percent,8,8)BTD(Port_Data.Data_Transfer[2],0,DFG2_DFG3.Write_Data.BDC1_Offset_Percent,0,8)BTD(Port_Data.Data_Transfer[3],0,DFG2_DFG3.Write_Data.BDC1_Teach_Selection,0,8)BTD(Port_Data.Data_Transfer[4],0,DFG2_DFG3.Write_Data.BDC1_Delay_Timer2,8,8)BTD(Port_Data.Data_Transfer[5],0,DFG2_DFG3.Write_Data.BDC1_Delay_Timer2,0,8)BTD(Port_Data.Data_Transfer[6],0,DFG2_DFG3.Write_Data.BDC1_Delay_Timer1,8,8)BTD(Port_Data.Data_Transfer[7],0,DFG2_DFG3.Write_Data.BDC1_Delay_Timer1,0,8)BTD(Port_Data.Data_Transfer[8],0,DFG2_DFG3.Write_Data.BDC1_Delay_Mode,0,8)OTU(Port_Data.Port_Read.[Port])OTL(Local_Control.6);
   46: NOP();
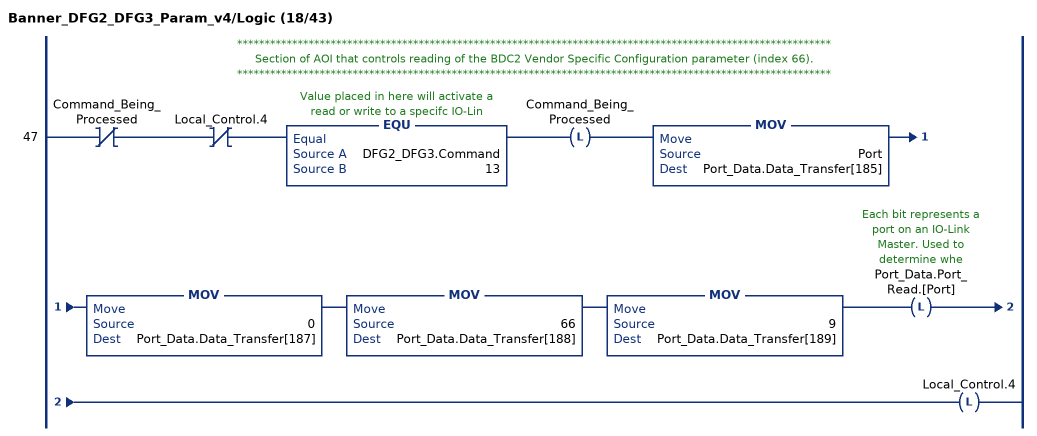
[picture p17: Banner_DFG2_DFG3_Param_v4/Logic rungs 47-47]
   // ************************************************************************************************************
   // Section of AOI that controls reading of the BDC2 Vendor Specific Configuration parameter (index 66).
   // ************************************************************************************************************
   47: XIO(Command_Being_Processed)XIO(Local_Control.4)EQU(DFG2_DFG3.Command,13)OTL(Command_Being_Processed)MOV(Port,Port_Data.Data_Transfer[185])MOV(0,Port_Data.Data_Transfer[187])MOV(66,Port_Data.Data_Transfer[188])MOV(9,Port_Data.Data_Transfer[189])OTL(Port_Data.Port_Read.[Port])OTL(Local_Control.4);
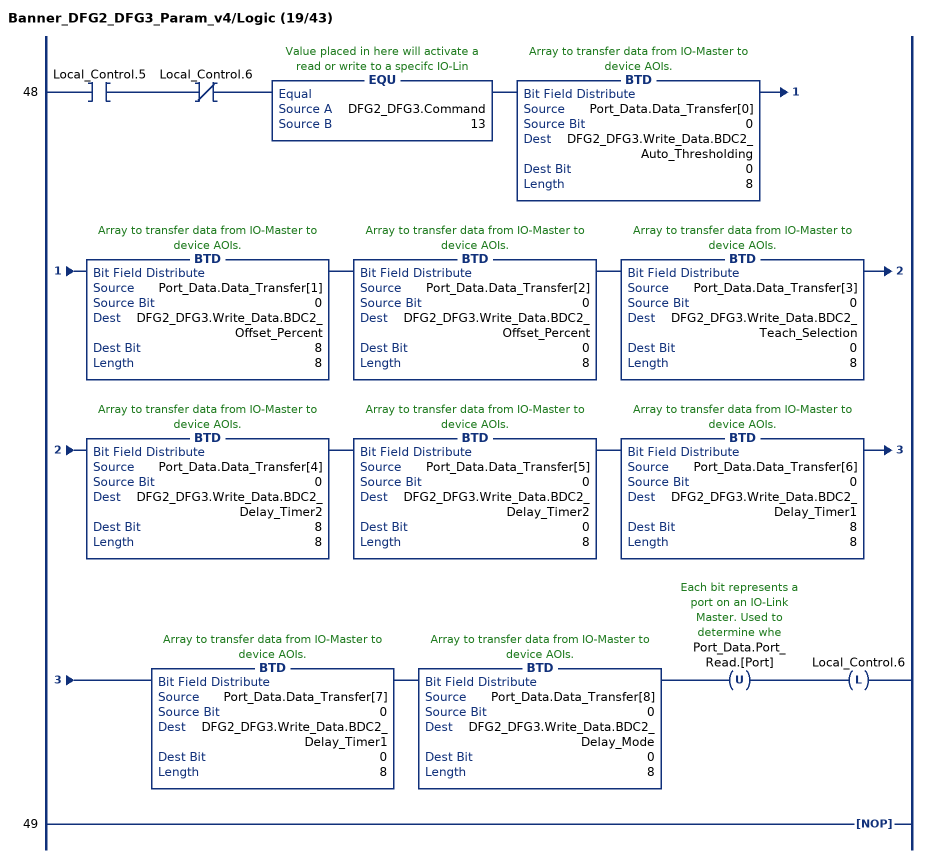
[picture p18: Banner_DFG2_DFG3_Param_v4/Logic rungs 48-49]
   48: XIC(Local_Control.5)XIO(Local_Control.6)EQU(DFG2_DFG3.Command,13)BTD(Port_Data.Data_Transfer[0],0,DFG2_DFG3.Write_Data.BDC2_Auto_Thresholding,0,8)BTD(Port_Data.Data_Transfer[1],0,DFG2_DFG3.Write_Data.BDC2_Offset_Percent,8,8)BTD(Port_Data.Data_Transfer[2],0,DFG2_DFG3.Write_Data.BDC2_Offset_Percent,0,8)BTD(Port_Data.Data_Transfer[3],0,DFG2_DFG3.Write_Data.BDC2_Teach_Selection,0,8)BTD(Port_Data.Data_Transfer[4],0,DFG2_DFG3.Write_Data.BDC2_Delay_Timer2,8,8)BTD(Port_Data.Data_Transfer[5],0,DFG2_DFG3.Write_Data.BDC2_Delay_Timer2,0,8)BTD(Port_Data.Data_Transfer[6],0,DFG2_DFG3.Write_Data.BDC2_Delay_Timer1,8,8)BTD(Port_Data.Data_Transfer[7],0,DFG2_DFG3.Write_Data.BDC2_Delay_Timer1,0,8)BTD(Port_Data.Data_Transfer[8],0,DFG2_DFG3.Write_Data.BDC2_Delay_Mode,0,8)OTU(Port_Data.Port_Read.[Port])OTL(Local_Control.6);
   49: NOP();
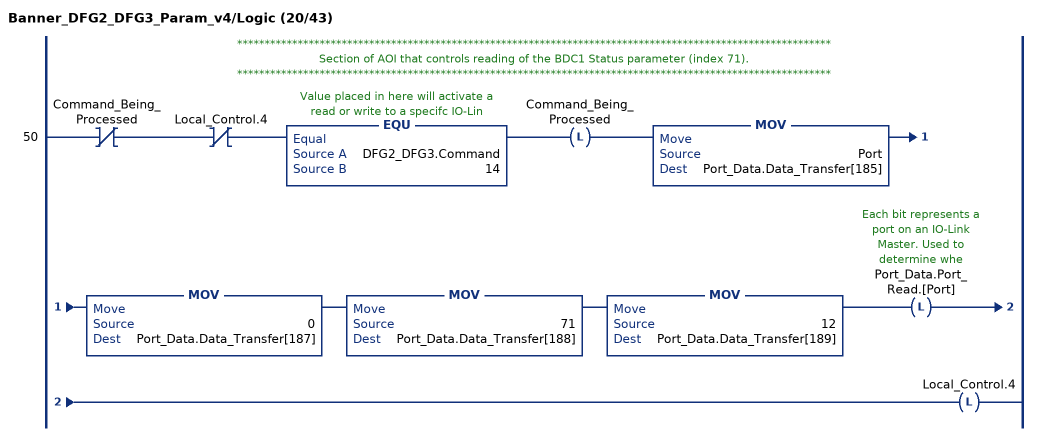
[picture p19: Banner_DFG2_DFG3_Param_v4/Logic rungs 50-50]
   // ************************************************************************************************************
   // Section of AOI that controls reading of the BDC1 Status parameter (index 71).
   // ************************************************************************************************************
   50: XIO(Command_Being_Processed)XIO(Local_Control.4)EQU(DFG2_DFG3.Command,14)OTL(Command_Being_Processed)MOV(Port,Port_Data.Data_Transfer[185])MOV(0,Port_Data.Data_Transfer[187])MOV(71,Port_Data.Data_Transfer[188])MOV(12,Port_Data.Data_Transfer[189])OTL(Port_Data.Port_Read.[Port])OTL(Local_Control.4);
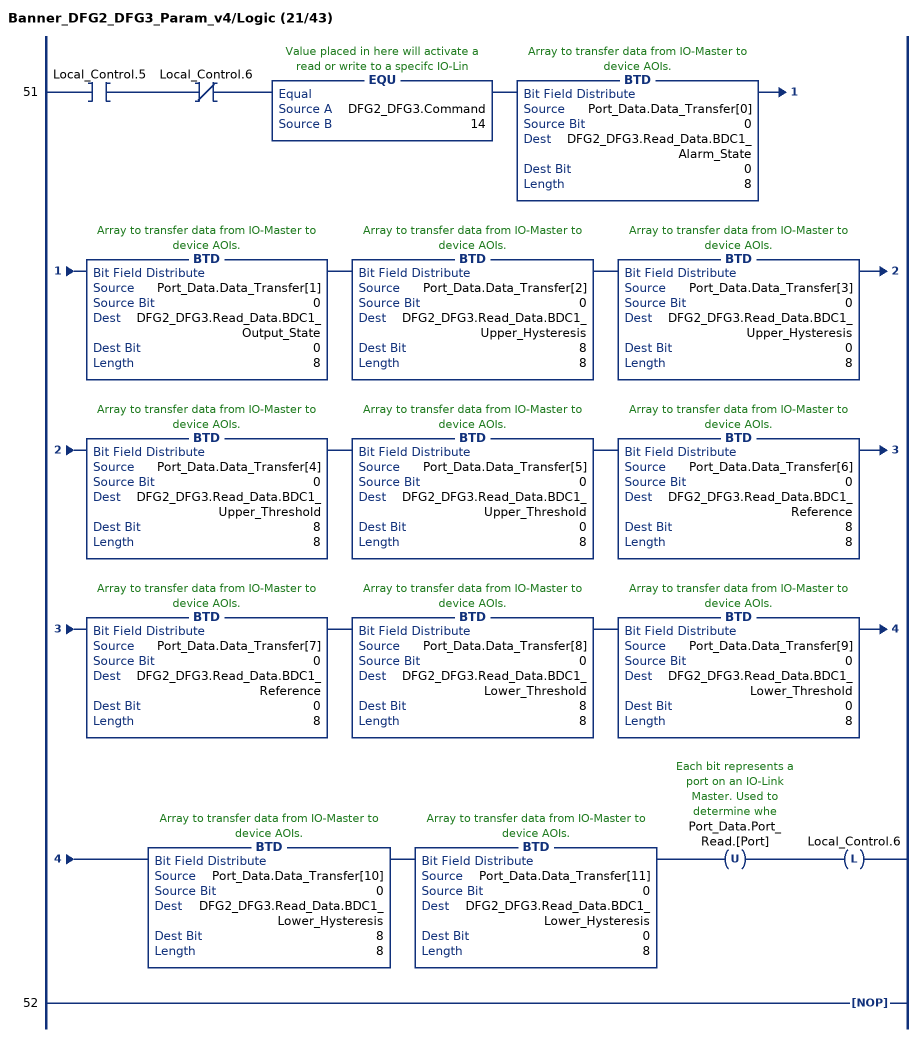
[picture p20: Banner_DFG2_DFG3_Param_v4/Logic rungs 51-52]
   51: XIC(Local_Control.5)XIO(Local_Control.6)EQU(DFG2_DFG3.Command,14)BTD(Port_Data.Data_Transfer[0],0,DFG2_DFG3.Read_Data.BDC1_Alarm_State,0,8)BTD(Port_Data.Data_Transfer[1],0,DFG2_DFG3.Read_Data.BDC1_Output_State,0,8)BTD(Port_Data.Data_Transfer[2],0,DFG2_DFG3.Read_Data.BDC1_Upper_Hysteresis,8,8)BTD(Port_Data.Data_Transfer[3],0,DFG2_DFG3.Read_Data.BDC1_Upper_Hysteresis,0,8)BTD(Port_Data.Data_Transfer[4],0,DFG2_DFG3.Read_Data.BDC1_Upper_Threshold,8,8)BTD(Port_Data.Data_Transfer[5],0,DFG2_DFG3.Read_Data.BDC1_Upper_Threshold,0,8)BTD(Port_Data.Data_Transfer[6],0,DFG2_DFG3.Read_Data.BDC1_Reference,8,8)BTD(Port_Data.Data_Transfer[7],0,DFG2_DFG3.Read_Data.BDC1_Reference,0,8)BTD(Port_Data.Data_Transfer[8],0,DFG2_DFG3.Read_Data.BDC1_Lower_Threshold,8,8)BTD(Port_Data.Data_Transfer[9],0,DFG2_DFG3.Read_Data.BDC1_Lower_Threshold,0,8)BTD(Port_Data.Data_Transfer[10],0,DFG2_DFG3.Read_Data.BDC1_Lower_Hysteresis,8,8)BTD(Port_Data.Data_Transfer[11],0,DFG2_DFG3.Read_Data.BDC1_Lower_Hysteresis,0,8)OTU(Port_Data.Port_Read.[Port])OTL(Local_Control.6);
   52: NOP();
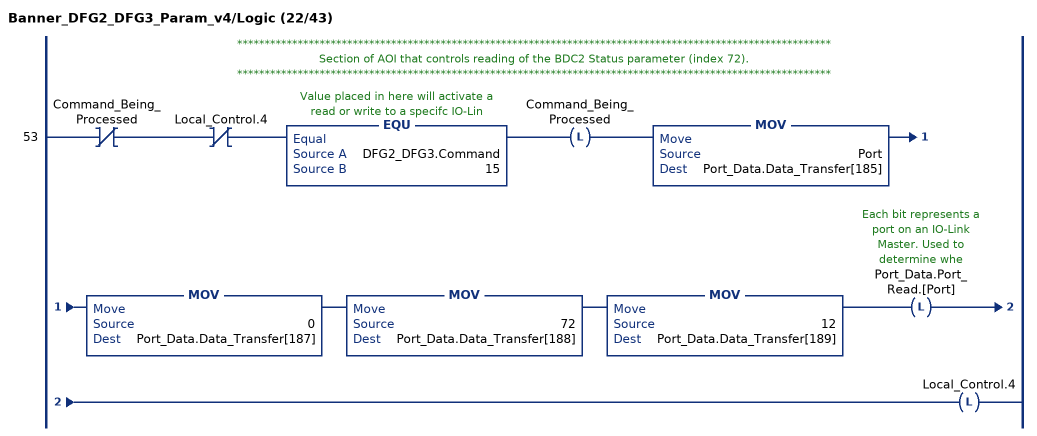
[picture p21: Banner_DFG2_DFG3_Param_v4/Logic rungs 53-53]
   // ************************************************************************************************************
   // Section of AOI that controls reading of the BDC2 Status parameter (index 72).
   // ************************************************************************************************************
   53: XIO(Command_Being_Processed)XIO(Local_Control.4)EQU(DFG2_DFG3.Command,15)OTL(Command_Being_Processed)MOV(Port,Port_Data.Data_Transfer[185])MOV(0,Port_Data.Data_Transfer[187])MOV(72,Port_Data.Data_Transfer[188])MOV(12,Port_Data.Data_Transfer[189])OTL(Port_Data.Port_Read.[Port])OTL(Local_Control.4);
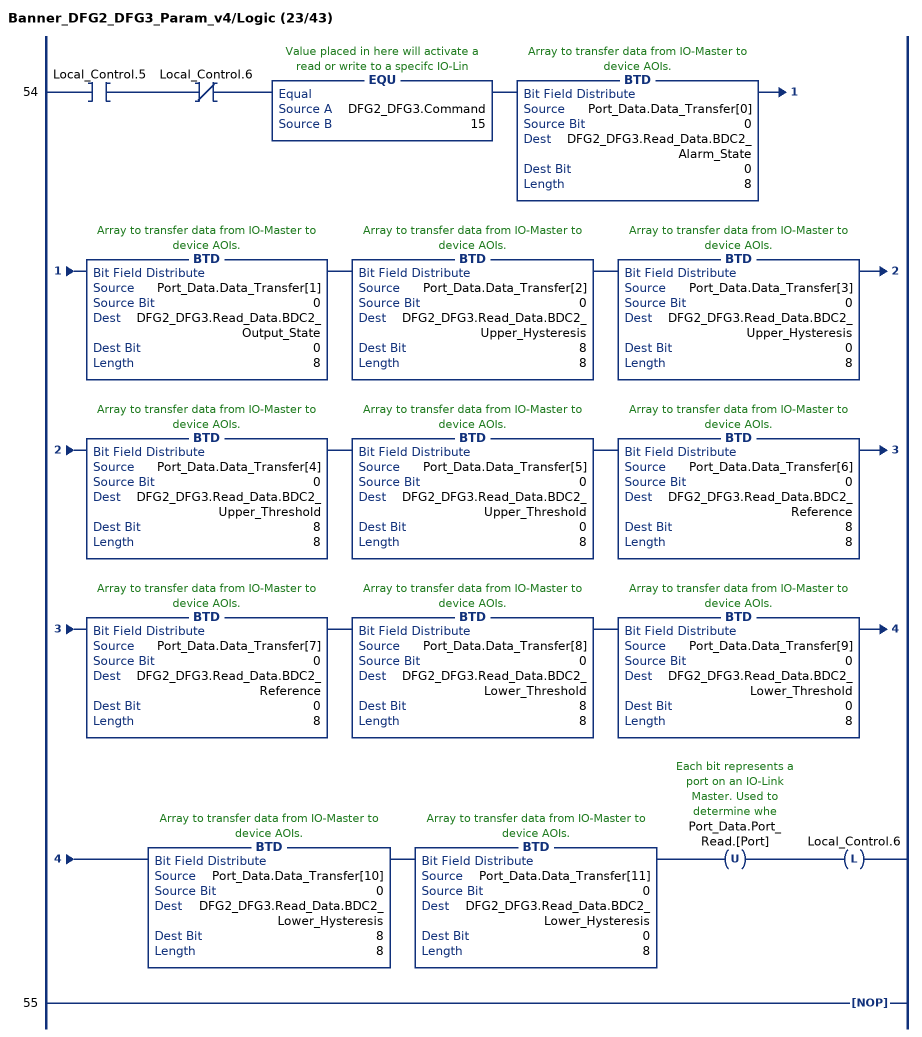
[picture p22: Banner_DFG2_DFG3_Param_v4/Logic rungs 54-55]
   54: XIC(Local_Control.5)XIO(Local_Control.6)EQU(DFG2_DFG3.Command,15)BTD(Port_Data.Data_Transfer[0],0,DFG2_DFG3.Read_Data.BDC2_Alarm_State,0,8)BTD(Port_Data.Data_Transfer[1],0,DFG2_DFG3.Read_Data.BDC2_Output_State,0,8)BTD(Port_Data.Data_Transfer[2],0,DFG2_DFG3.Read_Data.BDC2_Upper_Hysteresis,8,8)BTD(Port_Data.Data_Transfer[3],0,DFG2_DFG3.Read_Data.BDC2_Upper_Hysteresis,0,8)BTD(Port_Data.Data_Transfer[4],0,DFG2_DFG3.Read_Data.BDC2_Upper_Threshold,8,8)BTD(Port_Data.Data_Transfer[5],0,DFG2_DFG3.Read_Data.BDC2_Upper_Threshold,0,8)BTD(Port_Data.Data_Transfer[6],0,DFG2_DFG3.Read_Data.BDC2_Reference,8,8)BTD(Port_Data.Data_Transfer[7],0,DFG2_DFG3.Read_Data.BDC2_Reference,0,8)BTD(Port_Data.Data_Transfer[8],0,DFG2_DFG3.Read_Data.BDC2_Lower_Threshold,8,8)BTD(Port_Data.Data_Transfer[9],0,DFG2_DFG3.Read_Data.BDC2_Lower_Threshold,0,8)BTD(Port_Data.Data_Transfer[10],0,DFG2_DFG3.Read_Data.BDC2_Lower_Hysteresis,8,8)BTD(Port_Data.Data_Transfer[11],0,DFG2_DFG3.Read_Data.BDC2_Lower_Hysteresis,0,8)OTU(Port_Data.Port_Read.[Port])OTL(Local_Control.6);
   55: NOP();
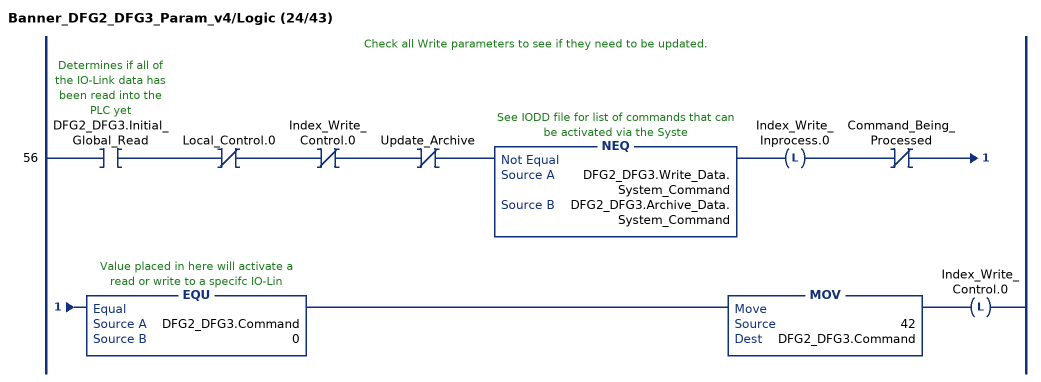
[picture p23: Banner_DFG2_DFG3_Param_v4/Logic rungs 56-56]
   // Check all Write parameters to see if they need to be updated.
   56: XIC(DFG2_DFG3.Initial_Global_Read)XIO(Local_Control.0)XIO(Index_Write_Control.0)XIO(Update_Archive)NEQ(DFG2_DFG3.Write_Data.System_Command,DFG2_DFG3.Archive_Data.System_Command)OTL(Index_Write_Inprocess.0)XIO(Command_Being_Processed)EQU(DFG2_DFG3.Command,0)MOV(42,DFG2_DFG3.Command)OTL(Index_Write_Control.0);
